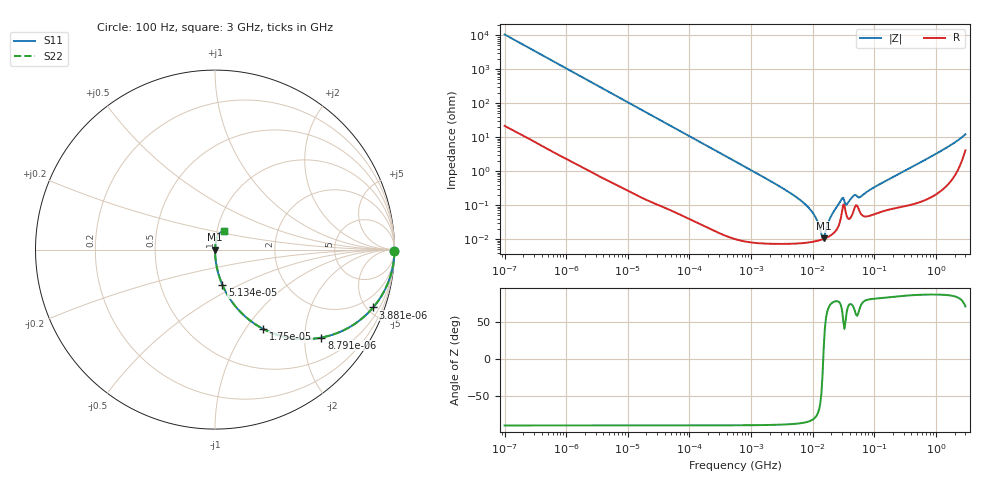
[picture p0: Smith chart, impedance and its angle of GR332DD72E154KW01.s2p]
!Murata Part Number: GR332DD72E154KW01
!These Parameters are Measured in Series Mode Connection
!Data Generated on Jun 10, 2025
!  o--ll--o
!Port1  Port2
!  o------o
!Operation Temp=25[degC], DC Bias Voltage=0[V]
!Freq. Start=100[Hz] Stop=3[GHz] 401[Steps]
# Hz S RI R 50
!Freq.(Hz) S11(Real) S11(Imag) S21(Real) S21(Imag) S12(Real) S12(Imag) S22(Real) S22(Imag)
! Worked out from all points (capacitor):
!   401 points, 100 Hz to 3 GHz, reference 50 ohm
!   read as one part in series: C = 151 nF near 109 Hz
!   lowest |Z| = 10.4 mohm at 15.06 MHz (marker M1)
!   series resonance near 14.81 MHz, so ESL is about 760 pH
!   S11 on the Smith chart (normalised r, x): 100 Hz: open; 3.881 kHz: 1.01, -5.46; 8.791 kHz: 1.01, -2.41; 17.5 kHz: 1.00, -1.21; 51.34 kHz: 1.00, -0.41; 3 GHz: 1.08, +0.23
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100  0.9999 -0.00948  0.000109 0.00948  0.000109 0.00948  0.9999 -0.00948
584  0.9968 -0.0551  0.00316 0.0551  0.00316 0.0551  0.9968 -0.0551
1788  0.9719 -0.1641  0.0281 0.1641  0.0281 0.1641  0.9719 -0.1641
3881  0.8812 -0.3224  0.1188 0.3224  0.1188 0.3224  0.8812 -0.3224
8791  0.5927 -0.4901  0.4073 0.4901  0.4073 0.4901  0.5927 -0.4901
17504  0.2696 -0.4424  0.7304 0.4424  0.7304 0.4424  0.2696 -0.4424
31977  0.1002 -0.2988  0.8998 0.2988  0.8998 0.2988  0.1002 -0.2988
51340  0.0418 -0.1985  0.9582 0.1985  0.9582 0.1985  0.0418 -0.1985
547723  0.000479 -0.0195  0.9995 0.0195  0.9995 0.0195  0.000479 -0.0195
4513443  7.73e-05 -0.00215  0.9999 0.00215  0.9999 0.00215  7.73e-05 -0.00215
7246509  7.78e-05 -0.00113  0.9999 0.00113  0.9999 0.00113  7.78e-05 -0.00113
9794414  8.27e-05 -0.000621  0.9999 0.000621  0.9999 0.000621  8.27e-05 -0.000621
1.163455e7  8.78e-05 -0.000357  0.9999 0.000357  0.9999 0.000357  8.78e-05 -0.000357
1.382041e7  9.57e-05 -0.000102  0.9999 0.000102  0.9999 0.000102  9.57e-05 -0.000102
1.506283e7  0.000101 2.5e-05  0.9999 -2.5e-05  0.9999 -2.5e-05  0.000101 2.5e-05
1.950129e7  0.000128 0.000426  0.9999 -0.000426  0.9999 -0.000426  0.000128 0.000426
2.872754e7  0.000431 0.00132  0.9996 -0.00132  0.9996 -0.00132  0.000431 0.00132
3.71925e7  0.000404 0.00109  0.9996 -0.00109  0.9996 -0.00109  0.000404 0.00109
4.612319e7  0.000681 0.00177  0.9993 -0.00177  0.9993 -0.00177  0.000681 0.00177
5.9714e7  0.000576 0.00166  0.9994 -0.00166  0.9994 -0.00166  0.000576 0.00166
1.751444e8  0.000772 0.00577  0.9992 -0.00577  0.9992 -0.00577  0.000772 0.00577
3e9  0.0507 0.1044  0.9493 -0.1044  0.9493 -0.1044  0.0507 0.1044
